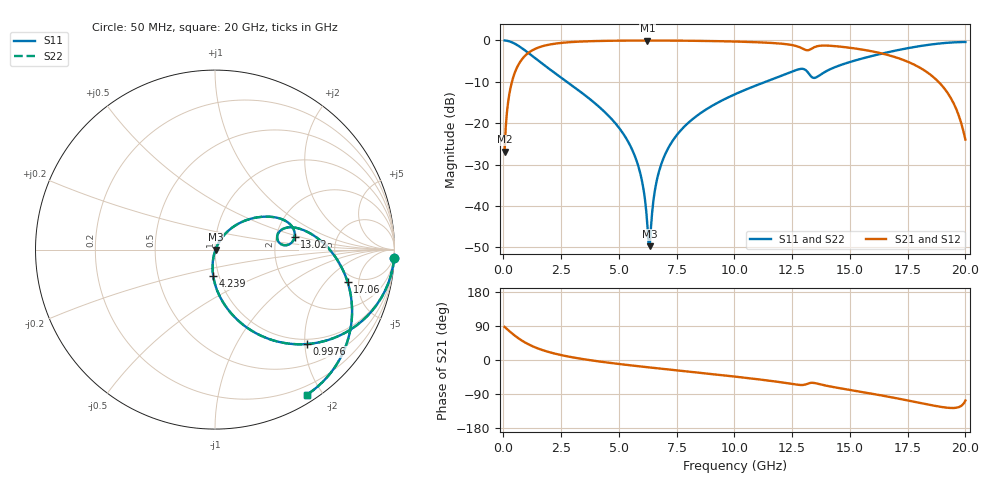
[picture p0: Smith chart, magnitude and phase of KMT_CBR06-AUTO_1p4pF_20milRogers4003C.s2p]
! Data measured by Modelithics Inc. support@modelithics.com 813-866-6335
! KEMET CBR06-AUTO 1.4pF, Pad Width= 0.851mm, Pad Length= 0.64mm, Pad Gap= 0.62mm, 20mil Rogers 4003C substrate Data, January 2022
# hz S ma R 50
! 2 Port Network Data from SP1.SP block
! freq  magS11  angS11  magS21  angS21  magS12  angS12  magS22  angS22
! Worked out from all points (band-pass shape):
!   401 points, 50 MHz to 20 GHz, reference 50 ohm
!   highest |S21| = -0.03 dB at 6.234 GHz (marker M1); lowest = -26.9 dB at 50 MHz (marker M2)
!   |S21| within 3 dB of the highest: 1.076 GHz to 16.29 GHz (15.21 GHz wide, 175 % of centre)
!   lowest |S11| = -49.7 dB at 6.334 GHz (marker M3), VSWR 1.01, Z = 50.3 + j0.0316 ohm
!   |S11| at or under -10 dB: 2.745 GHz to 11.35 GHz (8.604 GHz wide, 122 % of centre)
!   |S22| runs from -49.7 to 0.0 dB; largest |S21 - S12| = 0
!   S11 on the Smith chart (normalised r, x): 50 MHz: 1, -42; 997.6 MHz: 0.90, -2.05; 4.239 GHz: 0.94, -0.29; 13.02 GHz: 2.54, +0.44; 17.06 GHz: 4.15, -3.61; 20 GHz: 0.09, -1.81
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5e7  0.999 -2.7  0.04515 87.2  0.04515 87.2  0.999 -2.7
2.495e8  0.9753 -13.5  0.2203 76.5  0.2203 76.5  0.9753 -13.5
3.99125e8  0.94 -21.1  0.3403 68.8  0.3403 68.8  0.94 -21.1
9.97625e8  0.7345 -45.8  0.6773 44.1  0.6773 44.1  0.7345 -45.8
1.94525e9  0.4609 -68.4  0.8856 21.4  0.8856 21.4  0.4609 -68.4
3.391625e9  0.2327 -86.6  0.9702 2.9  0.9702 2.9  0.2327 -86.6
4.2395e9  0.1489 -93.7  0.9863 -4.6  0.9863 -4.6  0.1489 -93.7
5.685875e9  0.04026 -101.4  0.9962 -15.4  0.9962 -15.4  0.04026 -101.4
6.035e9  0.01768 -98.4  0.9968 -17.7  0.9968 -17.7  0.01768 -98.4
6.2345e9  0.005646 -77.9  0.9968 -19.1  0.9968 -19.1  0.005646 -77.9
6.33425e9  0.00326 5.5  0.9968 -19.7  0.9968 -19.7  0.00326 5.5
6.73325e9  0.026 60.9  0.9964 -22.4  0.9964 -22.4  0.026 60.9
7.780625e9  0.08793 58.6  0.9924 -29.1  0.9924 -29.1  0.08793 58.6
1.0025e10  0.2237 44.9  0.9695 -43.8  0.9695 -43.8  0.2237 44.9
1.30175e10  0.4489 8.9  0.7803 -65.5  0.7803 -65.5  0.4489 8.9
1.336662e10  0.3579 6.6  0.8023 -60.1  0.8023 -60.1  0.3579 6.6
1.456362e10  0.5 12.8  0.842 -74.5  0.842 -74.5  0.5 12.8
1.670825e10  0.7263 -9.6  0.6589 -97.4  0.6589 -97.4  0.7263 -9.6
1.705738e10  0.7617 -13.9  0.6154 -101.4  0.6154 -101.4  0.7617 -13.9
1.90025e10  0.9252 -41.3  0.2809 -124.3  0.2809 -124.3  0.9252 -41.3
1.955112e10  0.9491 -50.2  0.1601 -126.4  0.1601 -126.4  0.9491 -50.2
2e10  0.9568 -57.7  0.06328 -106.9  0.06328 -106.9  0.9568 -57.7
